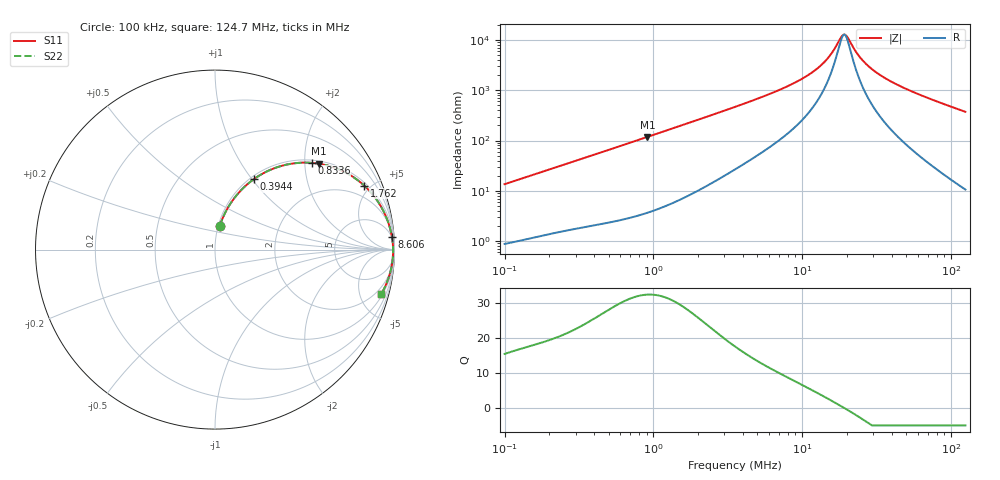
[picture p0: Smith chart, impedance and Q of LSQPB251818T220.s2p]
! LSQPB251818T220  S-PARAMETER MODEL  ( General Type )
! Model Generated by TAIYO YUDEN Corporation (http://www.ty-top.com)
! Version 2.0
! TAIYO YUDEN Control No. 100810NG19SB-FKC
! Copyright(c) 2009 TAIYO YUDEN CO.,LTD. All Rights Reserved.
! Product Description (link to TY-COMPAS)
! https://ds.yuden.co.jp/TYCOMPAS/or/detail?pn=LSQPB251818T220K&u=M
! Products Name : Inductors
! Characteristics :
!  Inductance : 22 uH , SRF(min) : 10 MHz , DC Resistance(max) : 0.728 Ohm
!  Rated Current : Saturation :640 mA , Temp Rise : 490 mA (40 degC)
!  Case Size : 2.5 x 1.8 / 0.098 x 0.071 [mm/inch] , Thickness : 1.8 / 0.071 [mm/inch]
!  (Conditions: Temperature = 25 degC , DC Bias Current/Voltage = 0A / 0V)
! External Node Assignments :
!  1  o---GGG---o  2
! GND o---------o GND
! Frequency Range : 0.1MHz  -  124.6553MHz  [ 402 STEP ]
# MHz S RI R 50
! Freq[MHz].  S11 Real  S11 Imag  S21 Real  S21 Imag  S12 Real  S12 Imag  S22 Real  S22 Imag
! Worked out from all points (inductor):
!   401 points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, 100 kHz to 124.7 MHz, reference 50 ohm
!   read as one part in series: L = 21.4 uH near 103.6 kHz
!   highest Q = 32.4 at 911.3 kHz (marker M1), where L = 20.6 uH
!   self-resonance near 18.85 MHz
!   S11 on the Smith chart (normalised r, x): 100 kHz: 1.02, +0.27; 394.4 kHz: 1.04, +1.03; 833.6 kHz: 1.07, +2.16; 1.762 MHz: 1.17, +4.58; 8.606 MHz: 4, +27; 124.7 MHz: 1.21, -7.47
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0.1  0.0261 0.1302  0.9739 -0.1302  0.9739 -0.1302  0.0261 0.1302
0.196831  0.0748 0.2385  0.9252 -0.2385  0.9252 -0.2385  0.0748 0.2385
0.330013  0.1681 0.3533  0.8319 -0.3533  0.8319 -0.3533  0.1681 0.3533
0.394389  0.2189 0.3943  0.7811 -0.3943  0.7811 -0.3943  0.2189 0.3943
0.594193  0.3776 0.4684  0.6224 -0.4684  0.6224 -0.4684  0.3776 0.4684
0.833631  0.5378 0.4833  0.4622 -0.4833  0.4622 -0.4833  0.5378 0.4833
0.911319  0.5802 0.4783  0.4198 -0.4783  0.4198 -0.4783  0.5802 0.4783
1.089088  0.6612 0.458  0.3388 -0.458  0.3388 -0.458  0.6612 0.458
1.762072  0.831 0.3571  0.169 -0.3571  0.169 -0.3571  0.831 0.3571
3.530656  0.9458 0.1997  0.0542 -0.1997  0.0542 -0.1997  0.9458 0.1997
8.606354  0.9856 0.0718  0.0144 -0.0718  0.0144 -0.0718  0.9856 0.0718
11.65164  0.9898 0.0423  0.0102 -0.0423  0.0102 -0.0423  0.9898 0.0423
14.68918  0.9915 0.022  0.00847 -0.022  0.00847 -0.022  0.9915 0.022
18.19151  0.9923 0.00416  0.00772 -0.00416  0.00772 -0.00416  0.9923 0.00416
19.19052  0.9923 -0.00025  0.00765 0.00025  0.00765 0.00025  0.9923 -0.00025
20.24438  0.9924 -0.00467  0.00762 0.00467  0.00762 0.00467  0.9924 -0.00467
23.34633  0.9922 -0.0166  0.00776 0.0166  0.00776 0.0166  0.9922 -0.0166
26.44805  0.9918 -0.0272  0.00815 0.0272  0.00815 0.0272  0.9918 -0.0272
31.04897  0.9909 -0.0416  0.00908 0.0416  0.00908 0.0416  0.9909 -0.0416
38.45196  0.9888 -0.0624  0.0112 0.0624  0.0112 0.0624  0.9888 -0.0624
63.33127  0.9773 -0.1227  0.0227 0.1227  0.0227 0.1227  0.9773 -0.1227
124.6553  0.9271 -0.2462  0.0729 0.2462  0.0729 0.2462  0.9271 -0.2462
